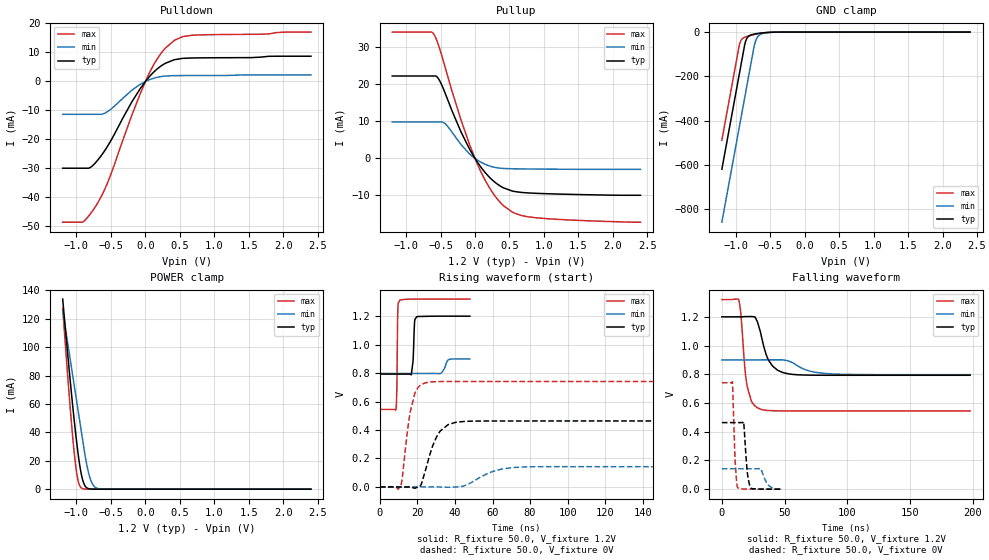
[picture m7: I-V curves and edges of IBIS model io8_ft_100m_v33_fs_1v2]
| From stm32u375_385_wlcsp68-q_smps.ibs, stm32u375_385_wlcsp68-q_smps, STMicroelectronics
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[Model]   io8_ft_100m_v33_fs_1v2
Model_type I/O
Polarity   Non-Inverting
Enable   Active-Low
| CAP_THRESHOLD on pad IOFT is "UDTCAPC" :
| Rising=30.0% of vddiom   Falling=70.0% of vddiom
| C_comp min and max val. don't necessarily correlate with the min and max pvt
| but are the smallest and greatest pad capacitance found.
| var   typ   min   max
C_comp   3.62609pF  3.42535pF  3.70436pF
|C_comp_pullup   2.21488pF  1.92185pF  2.35478pF
|C_comp_pulldown   1.41121pF  1.50350pF  1.34958pF
Vinl = 450.0mV
Vinh = 660.0mV
Vmeas = 600.0mV   | Reference voltage for timing measurements
Cref  = 50.0pF   | Timing specification test load capacitance value
Rref  = 1.0MOhm   | Timing specification test load resistance value
Vref  = 660.0mV   | Timing specification test load voltage
[Model Spec]
| TIME_THRESHOLD on pin ZIV33M is "CMOS" :
| Rising=50.0% of vddiom   Falling=50.0% of vddiom
Vinl 434.50000mV 327.50000mV 480.50000mV
Vinh 750.50000mV 549.50000mV 835.50000mV
| variable   typ   min   max
[Temperature Range] 25.0 130.0 -40.0
| variable   typ   min   max
[Voltage Range] 1.2V 900.0mV 1.32V
| variable   typ   min   max
[POWER Clamp Reference] 1.2V 900.0mV 1.32V
| variable   typ   min   max
[GND Clamp Reference] 0V 0V 0V
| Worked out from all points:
|   slope of the pulldown table from 0 to 0.18 V, typ, clamps not added: 40 ohm
|   slope of the pullup table from 0 to 0.18 V, typ, clamps not added: 40 ohm
|   GND clamp passes 1 mA (typ) near -0.50 V on its own axis
|   POWER clamp passes 1 mA (typ) near -0.85 V on its own axis
|   rising waveform, R_fixture 50.0, V_fixture 1.2V: 20-80 % time 754ps typ, 1.98ns min, 399ps max; typ from 0.793 V to 1.2 V
|   falling waveform, R_fixture 50.0, V_fixture 1.2V: 20-80 % time 9.11ns typ, 15.6ns min, 5ns max; typ from 1.2 V to 0.793 V
|   rising waveform, R_fixture 50.0, V_fixture 0V: 20-80 % time 7.27ns typ, 13.2ns min, 4.77ns max; typ from 0 V to 0.464 V
|   falling waveform, R_fixture 50.0, V_fixture 0V: 20-80 % time 2.5ns typ, 4.62ns min, 1.89ns max; typ from 0.464 V to 0 V
[POWER Clamp]
-1.2V     133.8mA    125.6mA    127.5mA
-1.08V    70.97mA    87.88mA    50.75mA
-1.04V    51.73mA    75.31mA    29.13mA
-1.01V    38.33mA    65.88mA    15.91mA
-970mV    22.56mA    53.3mA     4.74mA
-930mV    10.55mA    40.73mA    892.2uA
-890mV    3.611mA    28.15mA    138.3uA
-850mV    950.4uA    17.03mA    20.6uA
-810mV    222.1uA    8.794mA    3.05uA
-770mV    50.16uA    3.803mA    451.1nA
-650mV    561.7nA    165.6uA    1.537nA
2.4V      0A         0A         0A
[GND Clamp]
-1.2V     -620mA     -859.4mA   -488.5mA
-940mV    -178mA     -417.4mA   -50.52mA
-910mV    -127mA     -366.4mA   -31.92mA
-870mV    -59.03mA   -298.4mA   -23.56mA
-840mV    -30.06mA   -247.4mA   -20.12mA
-800mV    -16.5mA    -179.4mA   -16.42mA
-730mV    -9.175mA   -61.6mA    -10.9mA
-700mV    -7.461mA   -32.04mA   -8.862mA
-660mV    -5.584mA   -14.78mA   -6.456mA
-570mV    -2.482mA   -3.888mA   -2.491mA
-380mV    -62.94uA   -244.6uA   -21.21uA
2.4V      891.3pA    142.1nA    382.4pA
| variable   typ   min   max
[Pullup Reference] 1.2V 900.0mV 1.32V
| variable   typ   min   max
[Pulldown Reference] 0V 0V 0V
[Pullup]
-1.2V     22.28mA    9.872mA    34.14mA
-630mV    22.28mA    9.872mA    34.14mA
-600mV    22.28mA    9.872mA    33.65mA
-530mV    21.54mA    9.847mA    30.63mA
-430mV    17.48mA    9.347mA    24.42mA
-200mV    7.047mA    3.686mA    10.21mA
-10mV     299.4uA    135.1uA    455.2uA
200mV     -4.898mA   -1.964mA   -7.619mA
420mV     -8mA       -2.709mA   -12.87mA
580mV     -8.947mA   -2.8mA     -14.83mA
790mV     -9.331mA   -2.845mA   -15.82mA
2.4V      -9.943mA   -2.949mA   -17.22mA
[Pulldown]
-1.2V     -29.93mA   -11.33mA   -48.55mA
-910mV    -29.93mA   -11.33mA   -48.48mA
-810mV    -29.8mA    -11.33mA   -46.03mA
-710mV    -27.65mA   -11.33mA   -42.6mA
-620mV    -24.89mA   -11.22mA   -38.69mA
-530mV    -21.58mA   -10.08mA   -33.79mA
-200mV    -7.157mA   -3.075mA   -11.82mA
40mV      1.18mA     424.7uA    2.081mA
230mV     5.395mA    1.701mA    9.799mA
420mV     7.512mA    2.016mA    14.19mA
670mV     8.097mA    2.046mA    15.93mA
2.4V      8.706mA    2.25mA     17.03mA
[Ramp]
dV/dt_r 278.14112mV/7.22809ns 85.1975mV/13.03004ns 444.65493mV/4.52048ns
dV/dt_f 244.21047mV/8.82046ns 61.56275mV/15.56747ns 465.10837mV/4.84189ns
R_load = 50.0
| Removed startup time: 0s 0s 0s  .
| Removed end time: 47.95ns.
[Rising Waveform]
R_fixture   = 50.0
V_fixture   = 1.2V
V_fixture_min = 900.0mV
V_fixture_max = 1.32V
0s        793mV      797.4mV    544.8mV
8.55ns    793mV      797.4mV    542.8mV
9ns       793mV      797.4mV    670.6mV
9.6ns     793mV      797.4mV    1.257V
10.8ns    793mV      797.4mV    1.314V
16.75ns   788.5mV    797.4mV    1.319V
17.65ns   882.8mV    797.4mV    1.32V
18.55ns   1.167V     797.4mV    1.32V
19.6ns    1.196V     797.4mV    1.32V
47.95ns   1.2V       899.3mV    1.32V
| Removed startup time: 0s 0s 0s  .
| Removed end time: 197.95ns.
[Falling Waveform]
R_fixture   = 50.0
V_fixture   = 1.2V
V_fixture_min = 900.0mV
V_fixture_max = 1.32V
0s        1.2V       900mV      1.32V
13.4ns    1.2V       900mV      1.32V
15.05ns   1.2V       900mV      1.227V
20.2ns    1.202V     900mV      714.1mV
26.45ns   1.198V     900mV      578.5mV
30.6ns    1.1V       900mV      557.9mV
37.4ns    895.5mV    900.5mV    547.5mV
52.55ns   803.8mV    894.7mV    544.9mV
84.85ns   793.1mV    804.1mV    544.8mV
197.9ns   793mV      797.4mV    544.8mV
| Removed startup time: 0s 0s 0s  .
| Removed end time: 197.9ns.
[Rising Waveform]
R_fixture   = 50.0
V_fixture   = 0V
V_fixture_min = 0V
V_fixture_max = 0V
0s        4.987nV    173.7nV    3.506nV
11.15ns   -12.68nV   173.4nV    9.093mV
16.15ns   119.4uV    167.9nV    525.5mV
18.75ns   -8.803mV   149.2nV    661.4mV
21.7ns    11.09mV    1.137uV    715.9mV
24.25ns   115.3mV    1.061uV    731.5mV
31ns      370.5mV    39.01uV    740.1mV
40.4ns    454mV      -102.9uV   741mV
72.7ns    463.5mV    137.7mV    741.1mV
197.9ns   463.6mV    142mV      741.1mV
| Removed startup time: 0s 0s 0s  .
| Removed end time: 47.95ns.
[Falling Waveform]
R_fixture   = 50.0
V_fixture   = 0V
V_fixture_min = 0V
V_fixture_max = 0V
0s        463.6mV    142mV      741.1mV
8.35ns    463.6mV    142mV      748.4mV
10.65ns   463.6mV    142mV      189.8mV
12.75ns   463.6mV    142mV      9.665mV
17.35ns   468.8mV    142mV      1.105mV
20.3ns    116.1mV    142mV      445.7uV
22.55ns   13.61mV    142mV      246.8uV
30.65ns   770.9uV    145.1mV    34.21uV
37.2ns    238.8uV    26.71mV    7.323uV
47.95ns   66.89uV    1.422mV    589.1nV
